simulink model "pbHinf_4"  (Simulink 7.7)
settings: Solver=ode45  StartTime=0.0  StopTime=10.0  RelTol=1e-3
libraries: cstblocks x1

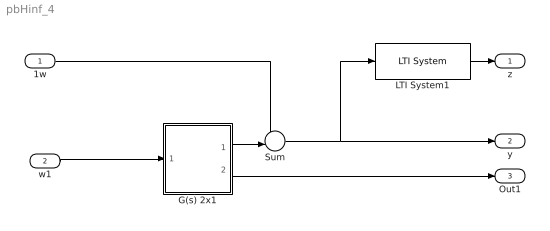
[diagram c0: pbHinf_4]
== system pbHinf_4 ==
  1w : Inport
  w1 : Inport  Port=2
  G(s) 2x1 : Subsystem
  LTI System1 : cstblocks/LTI System  SystemSampleTime=-1  sys=W1  IC=[]
  Sum : Sum  Inputs=+-|
  z : Outport
  y : Outport  Port=2
  Out1 : Outport  Port=3
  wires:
  1w/1 -> Sum/1
  LTI System1/1 -> z/1
  Sum/1 -> LTI System1/1, y/1
  w1/1 -> G(s) 2x1/1(u)
  G(s) 2x1/1(Position) -> Sum/2
  G(s) 2x1/2(Vitesse) -> Out1/1

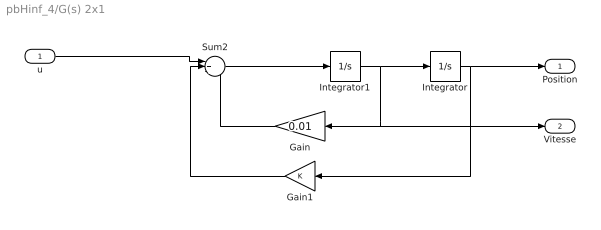
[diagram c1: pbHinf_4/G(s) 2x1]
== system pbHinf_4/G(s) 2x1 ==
  u : Inport
  Gain : Gain  Gain=0.01
  Gain1 : Gain
  Integrator : Integrator
  Integrator1 : Integrator
  Sum2 : Sum  Inputs=|+--
  Position : Outport
  Vitesse : Outport  Port=2
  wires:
  Gain1/1 -> Sum2/2
  Gain/1 -> Sum2/3
  Integrator1/1 -> Integrator/1, Gain/1, Vitesse/1
  Integrator/1 -> Gain1/1, Position/1
  Sum2/1 -> Integrator1/1
  u/1 -> Sum2/1
